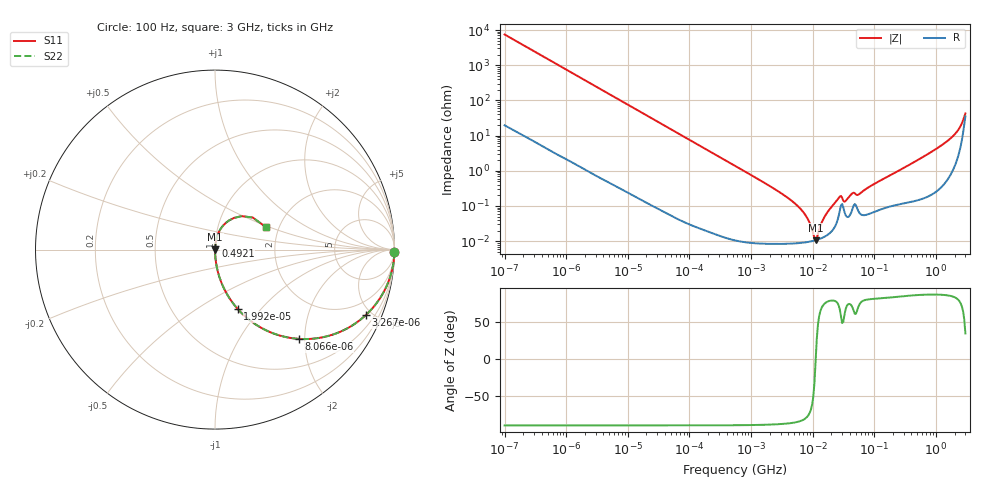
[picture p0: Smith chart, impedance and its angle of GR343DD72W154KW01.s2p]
!Murata Part Number: GR343DD72W154KW01
!These Parameters are Measured in Series Mode Connection
!Data Generated on Mar 13, 2026
!  o--ll--o
!Port1  Port2
!  o------o
!Operation Temp=25[degC], DC Bias Voltage=0[V]
!Freq. Start=100[Hz] Stop=3[GHz] 401[Steps]
# Hz S RI R 50
!Freq.(Hz) S11(Real) S11(Imag) S21(Real) S21(Imag) S12(Real) S12(Imag) S22(Real) S22(Imag)
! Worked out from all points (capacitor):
!   401 points, 100 Hz to 3 GHz, reference 50 ohm
!   read as one part in series: C = 213 nF near 109 Hz
!   lowest |Z| = 10.6 mohm at 11.14 MHz (marker M1)
!   series resonance near 11.18 MHz, so ESL is about 950 pH
!   S11 on the Smith chart (normalised r, x): 100 Hz: open; 3.267 kHz: 1.01, -4.61; 8.066 kHz: 1.01, -1.87; 19.92 kHz: 1.00, -0.76; 492.1 MHz: 1.00, +0.04; 3 GHz: 1.70, +0.48
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100  0.9998 -0.0134  0.000214 0.0134  0.000214 0.0134  0.9998 -0.0134
536  0.9947 -0.071  0.00526 0.071  0.00526 0.071  0.9947 -0.071
1788  0.9459 -0.2247  0.0541 0.2247  0.0541 0.2247  0.9459 -0.2247
3267  0.8408 -0.3644  0.1592 0.3644  0.1592 0.3644  0.8408 -0.3644
8066  0.4666 -0.4973  0.5334 0.4973  0.5334 0.4973  0.4666 -0.4973
19917  0.1266 -0.3309  0.8734 0.3309  0.8734 0.3309  0.1266 -0.3309
31977  0.0537 -0.2236  0.9463 0.2236  0.9463 0.2236  0.0537 -0.2236
547723  0.000296 -0.0138  0.9997 0.0138  0.9997 0.0138  0.000296 -0.0138
4919190  8.71e-05 -0.00125  0.9999 0.00125  0.9999 0.00125  8.71e-05 -0.00125
7565221  9.22e-05 -0.000549  0.9999 0.000549  0.9999 0.000549  9.22e-05 -0.000549
9794414  9.97e-05 -0.000183  0.9999 0.000183  0.9999 0.000183  9.97e-05 -0.000183
1.11444e7  0.000106 -4.9e-06  0.9999 4.9e-06  0.9999 4.9e-06  0.000106 -4.9e-06
1.572531e7  0.000135 0.000491  0.9999 -0.000491  0.9999 -0.000491  0.000135 0.000491
2.635803e7  0.000524 0.0016  0.9995 -0.0016  0.9995 -0.0016  0.000524 0.0016
3.412477e7  0.000547 0.00127  0.9995 -0.00127  0.9995 -0.00127  0.000547 0.00127
4.418008e7  0.000828 0.00215  0.9992 -0.00215  0.9992 -0.00215  0.000828 0.00215
5.719833e7  0.000637 0.00209  0.9994 -0.00209  0.9994 -0.00209  0.000637 0.00209
1.751444e8  0.001 0.00716  0.999 -0.00716  0.999 -0.00716  0.001 0.00716
4.920662e8  0.00181 0.0195  0.9982 -0.0195  0.9982 -0.0195  0.00181 0.0195
1.71441e9  0.0141 0.0804  0.9859 -0.0804  0.9859 -0.0804  0.0141 0.0804
2.419119e9  0.059 0.1478  0.941 -0.1478  0.941 -0.1478  0.059 0.1478
3e9  0.282 0.1265  0.718 -0.1265  0.718 -0.1265  0.282 0.1265
